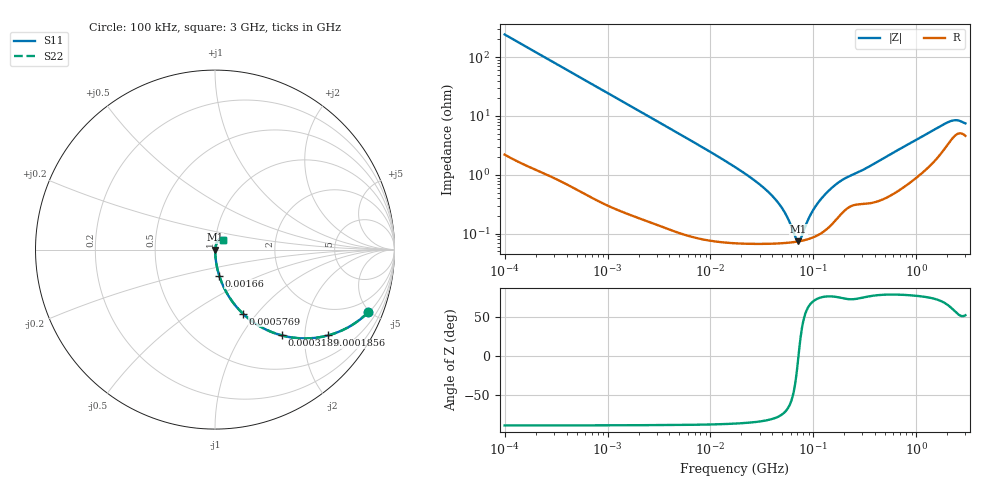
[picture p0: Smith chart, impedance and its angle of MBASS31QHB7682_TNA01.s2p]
! MBASS31QHB7682_TNA01  S-PARAMETER MODEL  ( Standard Model )
! Model Generated by TAIYO YUDEN Corporation (http://www.ty-top.com)
! Version 1.0
! TAIYO YUDEN Control No. 220601
! Copyright(c) 2013 TAIYO YUDEN CO.,LTD. All Rights Reserved.
! Product Description (link to TY-COMPAS)
! https://ds.yuden.co.jp/TYCOMPAS/or/detail?pn=MBASS31QHB7682KTNA01&u=M
! Products Name : Multilayer Ceramic Capacitors
! Characteristics :
!  Capacitance : 6800 [pF] , Rated Voltage : 630 [V] , TCC : X7R
!  Case Size : 3.2 x 1.6 / 0.126 x 0.063 [mm/inch] , Thickness : 1.15 / 0.045 [mm/inch]
!  (Conditions: Temperature = 25 [degC] , DC Bias Voltage = 0 [V])
! External Node Assignments :
!  1  o---| |---o  2
! GND o---------o GND
! Frequency Range : 100kHz  -  3GHz  [ 401 STEP ]
# MHZ S RI R 50
! Freq[MHz].  S11 Real  S11 Imag  S21 Real  S21 Imag  S12 Real  S12 Imag  S22 Real  S22 Imag
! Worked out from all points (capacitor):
!   401 points, 100 kHz to 3 GHz, reference 50 ohm
!   read as one part in series: C = 6.56 nF near 105.3 kHz
!   lowest |Z| = 74.1 mohm at 71.48 MHz (marker M1)
!   series resonance near 71.73 MHz, so ESL is about 750 pH
!   S11 on the Smith chart (normalised r, x): 100 kHz: 1.04, -4.85; 185.6 kHz: 1.03, -2.62; 318.9 kHz: 1.02, -1.53; 576.9 kHz: 1.01, -0.85; 1.66 MHz: 1.00, -0.30; 3 GHz: 1.09, +0.12
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0.1  0.8523 -0.3503  0.1477 0.3503  0.1477 0.3503  0.8523 -0.3503
0.185621  0.6304 -0.4778  0.3696 0.4778  0.3696 0.4778  0.6304 -0.4778
0.318916  0.3705 -0.4775  0.6295 0.4775  0.6295 0.4775  0.3705 -0.4775
0.562235  0.1624 -0.3631  0.8376 0.3631  0.8376 0.3631  0.1624 -0.3631
0.576913  0.1557 -0.3568  0.8443 0.3568  0.8443 0.3568  0.1557 -0.3568
0.917447  0.0695 -0.2484  0.9305 0.2484  0.9305 0.2484  0.0695 -0.2484
1.659646  0.0235 -0.1447  0.9765 0.1447  0.9765 0.1447  0.0235 -0.1447
3.161081  0.00743 -0.0776  0.9926 0.0776  0.9926 0.0776  0.00743 -0.0776
17.7727  0.000859 -0.0132  0.9991 0.0132  0.9991 0.0132  0.000859 -0.0132
29.75839  0.000719 -0.00695  0.9993 0.00695  0.9993 0.00695  0.000719 -0.00695
42.68829  0.000694 -0.00379  0.9993 0.00379  0.9993 0.00379  0.000694 -0.00379
52.46276  0.000699 -0.00222  0.9993 0.00222  0.9993 0.00222  0.000699 -0.00222
67.88584  0.00073 -0.000386  0.9993 0.000386  0.9993 0.000386  0.00073 -0.000386
71.47675  0.00074 -2.42e-05  0.9993 2.42e-05  0.9993 2.42e-05  0.00074 -2.42e-05
75.25761  0.000753 0.000339  0.9992 -0.000339  0.9992 -0.000339  0.000753 0.000339
97.38194  0.000858 0.0022  0.9991 -0.0022  0.9991 -0.0022  0.000858 0.0022
126.0104  0.00111 0.00425  0.9989 -0.00425  0.9989 -0.00425  0.00111 0.00425
171.6802  0.00189 0.00697  0.9981 -0.00697  0.9981 -0.00697  0.00189 0.00697
547.5153  0.00476 0.0212  0.9952 -0.0212  0.9952 -0.0212  0.00476 0.0212
2038.117  0.0369 0.0663  0.9631 -0.0663  0.9631 -0.0663  0.0369 0.0663
2441.062  0.0501 0.0634  0.9499 -0.0634  0.9499 -0.0634  0.0501 0.0634
3000  0.047 0.0537  0.953 -0.0537  0.953 -0.0537  0.047 0.0537
